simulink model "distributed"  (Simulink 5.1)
settings: Solver=ode45  StartTime=0.0  StopTime=0.6  RelTol=1e-3
InitFcn:
  | clear functions
libraries: truetime x5, simulink x1

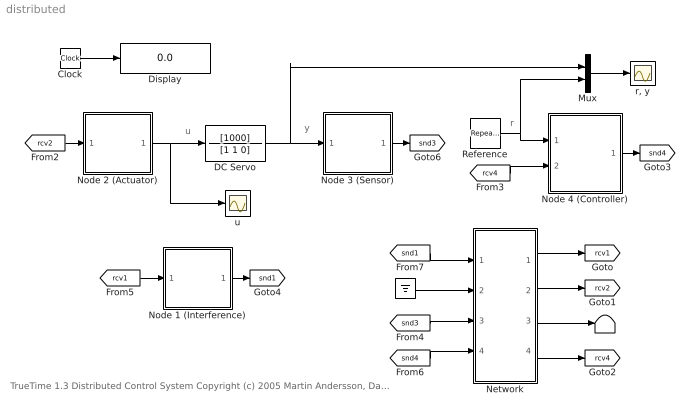
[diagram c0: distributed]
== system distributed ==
  note: u
  note: y
  note: r
  note: TrueTime 1.3 Distributed Control System Copyright (c) 2005 Martin Andersson, Dan Henriksson and Anton Cervin Department of Automatic Control, Lund University, Sweden Please direct questions and bug reports to: truetime@control.lth.se
  " " : Ground
  "       " : Terminator
  Clock : Clock
  DC Servo : TransferFcn  Numerator=[1000]  Denominator=[1 1 0]  AbsoluteTolerance=auto  Realization=auto
  Display : Display
  Mux : Mux  Inputs=2
  Network : Subsystem  SimViewingDevice=off
  Node 1 (Interference) : Subsystem  SimViewingDevice=off
  Node 2 (Actuator) : Subsystem  SimViewingDevice=off
  Node 3 (Sensor) : Subsystem  SimViewingDevice=off
  Node 4 (Controller) : Subsystem  SimViewingDevice=off
  Reference : simulink/Sources/Repeating Sequence  rep_seq_t=[0 0.3 0.3 0.6]  rep_seq_y=[1 1 0 0]
  "r, y" : Scope
  u : Scope
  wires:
  [snd1] -> Network/1(snd1)
  " "/1 -> Network/2(snd2)
  Network/1(rcv1) -> [rcv1]
  Node 2 (Actuator)/1(D/A) -> DC Servo/1, u/1
  Node 4 (Controller)/1(Snd) -> [snd4]
  [rcv2] -> Node 2 (Actuator)/1(Rcv)
  Clock/1 -> Display/1
  Reference/1 -> Node 4 (Controller)/1(AI1), Mux/2
  Network/2(rcv2) -> [rcv2]
  [rcv4] -> Node 4 (Controller)/2(Rcv)
  Mux/1 -> "r, y"/1
  Node 1 (Interference)/1(Snd) -> [snd1]
  Network/3(rcv3) -> "       "/1
  [snd3] -> Network/3(snd3)
  [rcv1] -> Node 1 (Interference)/1(Rcv)
  DC Servo/1 -> Node 3 (Sensor)/1(A/D), Mux/1
  Node 3 (Sensor)/1(Snd) -> [snd3]
  Network/4(rcv4) -> [rcv4]
  [snd4] -> Network/4(snd4)

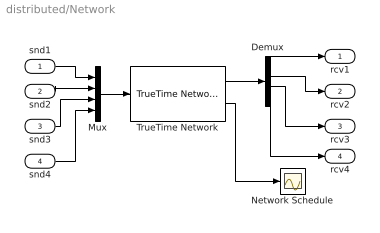
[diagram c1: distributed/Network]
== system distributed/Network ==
  snd1 : Inport  Port=1  PortDimensions=-1  SampleTime=-1  DataType=auto
  snd2 : Inport  Port=2  PortDimensions=-1  SampleTime=-1  DataType=auto
  snd3 : Inport  Port=3  PortDimensions=-1  SampleTime=-1  DataType=auto
  snd4 : Inport  Port=4  PortDimensions=-1  SampleTime=-1  DataType=auto
  Demux : Demux  Outputs=4  BusSelectionMode=off
  Mux : Mux  Inputs=4
  Network Schedule : Scope
  TrueTime Network : truetime/TrueTime Network  nwtype=CSMA/AMP (CAN)  nwnbr=1  nnodes=4  rate=80000  minsize=5  lossprob=0  bandwidths=1  slotsize=20  schedule="[1 2 3  3 3 3]"  memsize=10000  buftype=Common buffer  overflow=Retransmit
  rcv1 : Outport  Port=1
  rcv2 : Outport  Port=2
  rcv3 : Outport  Port=3
  rcv4 : Outport  Port=4
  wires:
  Demux/1 -> rcv1/1
  Demux/2 -> rcv2/1
  Mux/1 -> TrueTime Network/1
  snd1/1 -> Mux/1
  snd2/1 -> Mux/2
  snd3/1 -> Mux/3
  Demux/3 -> rcv3/1
  snd4/1 -> Mux/4
  Demux/4 -> rcv4/1
  TrueTime Network/1 -> Demux/1
  TrueTime Network/2 -> Network Schedule/1

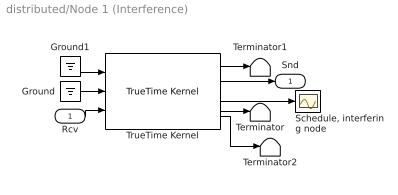
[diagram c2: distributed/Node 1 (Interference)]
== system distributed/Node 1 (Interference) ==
  Rcv : Inport  Port=1  PortDimensions=-1  SampleTime=-1  DataType=auto
  Ground : Ground
  Ground1 : Ground
  "Schedule, interfering node" : Scope
  Terminator : Terminator
  Terminator1 : Terminator
  Terminator2 : Terminator
  TrueTime Kernel : truetime/TrueTime Kernel  sfun=interference_init  args=0  battery=off  clockdrift=0  clockoffset=0
  Snd : Outport  Port=1
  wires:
  TrueTime Kernel/3 -> "Schedule, interfering node"/1
  TrueTime Kernel/2 -> Snd/1
  TrueTime Kernel/1 -> Terminator1/1
  Ground/1 -> TrueTime Kernel/2
  Rcv/1 -> TrueTime Kernel/3
  Ground1/1 -> TrueTime Kernel/1
  TrueTime Kernel/4 -> Terminator/1
  TrueTime Kernel/5 -> Terminator2/1

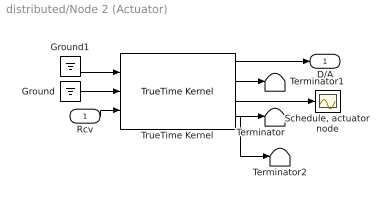
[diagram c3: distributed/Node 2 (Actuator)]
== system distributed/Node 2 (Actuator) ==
  Rcv : Inport  Port=1  PortDimensions=-1  SampleTime=-1  DataType=auto
  Ground : Ground
  Ground1 : Ground
  "Schedule, actuator node" : Scope
  Terminator : Terminator
  Terminator1 : Terminator
  Terminator2 : Terminator
  TrueTime Kernel : truetime/TrueTime Kernel  sfun=actuator_init  args=0  battery=off  clockdrift=0  clockoffset=0
  D/A : Outport  Port=1
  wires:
  Ground1/1 -> TrueTime Kernel/1
  Rcv/1 -> TrueTime Kernel/3
  Ground/1 -> TrueTime Kernel/2
  TrueTime Kernel/1 -> D/A/1
  TrueTime Kernel/2 -> Terminator1/1
  TrueTime Kernel/3 -> "Schedule, actuator node"/1
  TrueTime Kernel/4 -> Terminator/1
  TrueTime Kernel/5 -> Terminator2/1

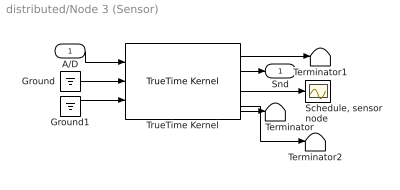
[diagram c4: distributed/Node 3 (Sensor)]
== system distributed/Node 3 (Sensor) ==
  A/D : Inport  Port=1  PortDimensions=-1  SampleTime=-1  DataType=auto
  Ground : Ground
  Ground1 : Ground
  "Schedule, sensor node" : Scope
  Terminator : Terminator
  Terminator1 : Terminator
  Terminator2 : Terminator
  TrueTime Kernel : truetime/TrueTime Kernel  sfun=sensor_init  args=0  battery=off  clockdrift=0  clockoffset=0
  Snd : Outport  Port=1
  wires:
  TrueTime Kernel/4 -> Terminator/1
  TrueTime Kernel/3 -> "Schedule, sensor node"/1
  TrueTime Kernel/2 -> Snd/1
  TrueTime Kernel/1 -> Terminator1/1
  Ground/1 -> TrueTime Kernel/2
  Ground1/1 -> TrueTime Kernel/3
  A/D/1 -> TrueTime Kernel/1
  TrueTime Kernel/5 -> Terminator2/1

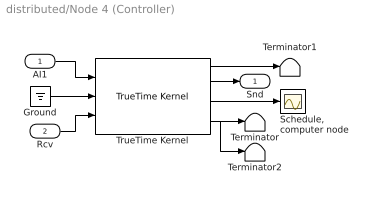
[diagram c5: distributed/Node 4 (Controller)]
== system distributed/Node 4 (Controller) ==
  AI1 : Inport  Port=1  PortDimensions=-1  SampleTime=-1  DataType=auto
  Rcv : Inport  Port=2  PortDimensions=-1  SampleTime=-1  DataType=auto
  Ground : Ground
  "Schedule, computer node" : Scope
  Terminator : Terminator
  Terminator1 : Terminator
  Terminator2 : Terminator
  TrueTime Kernel : truetime/TrueTime Kernel  sfun=controller_init  args=0  battery=off  clockdrift=0  clockoffset=0
  Snd : Outport  Port=1
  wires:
  TrueTime Kernel/2 -> Snd/1
  Ground/1 -> TrueTime Kernel/2
  AI1/1 -> TrueTime Kernel/1
  Rcv/1 -> TrueTime Kernel/3
  TrueTime Kernel/3 -> "Schedule, computer node"/1
  TrueTime Kernel/1 -> Terminator1/1
  TrueTime Kernel/4 -> Terminator/1
  TrueTime Kernel/5 -> Terminator2/1
